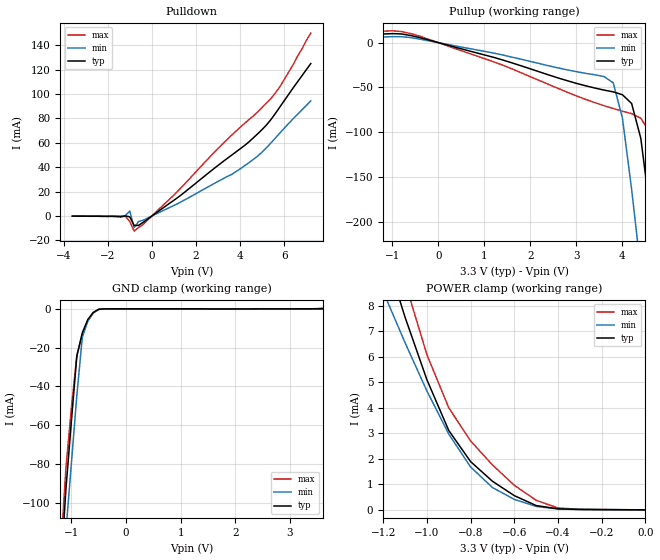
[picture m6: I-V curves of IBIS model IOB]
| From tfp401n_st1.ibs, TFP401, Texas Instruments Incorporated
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|   INPUT / OUTPUT  MODEL
[Model]   IOB
Model_type   I/O
| Signals   CTL1, CTL2, CTL3, SCDT
Vinl = 1.08
Vinh = 2.10
| variable   typ   min   max
C_comp   2pF   NA   NA
|   typ   min   max
[Temperature Range] 25.0   70.0   0.0
[Voltage range]   3.3V   3.0V   3.6V
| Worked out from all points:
|   slope of the pulldown table from 0 to 0.495 V, typ, clamps not added: 76.7 ohm
|   slope of the pullup table from 0 to 0.495 V, typ, clamps not added: 72.2 ohm
|   GND clamp passes 1 mA (typ) near -0.55 V on its own axis
|   POWER clamp passes 1 mA (typ) near -0.68 V on its own axis
[GND_clamp]
|Voltage   I(typ)   I(min)   I(max)
-3.6V     -1.31A     -1.33A     -1.29A
-1.2V     -138mA     -161mA     -127mA
-1.1V     -93mA      -115mA     -82.2mA
-1V       -58mA      -79.8mA    -51.2mA
-900mV    -24.3mA    -44.7mA    -24.1mA
-800mV    -12.4mA    -14.8mA    -13.4mA
-700mV    -5.53mA    -6.32mA    -6.36mA
-600mV    -1.83mA    -2.13mA    -2.17mA
-500mV    -221uA     -304uA     -325uA
3.3V      5.05nA     13.8uA     -16.9uA
3.6V      15.8uA     402uA      272pA
[Power_clamp]
|Note that the [Power_clamp] voltage table is referenced to Vcc
|and is calculated using Vtable=Vcc-Vmeasured.
|Voltage   I(typ)   I(min)   I(max)
-3.3V     76.1mA     54.4mA     97mA
-1.2V     10.3mA     8.55mA     12.2mA
-1.1V     7.55mA     6.55mA     8.92mA
-1V       5.1mA      4.66mA     6.08mA
-900mV    3.11mA     2.97mA     4mA
-800mV    1.89mA     1.68mA     2.7mA
-700mV    1.12mA     874uA      1.76mA
-600mV    557uA      410uA      963uA
-500mV    168uA      135uA      373uA
-400mV    40.3uA     33.2uA     73.3uA
-300mV    15.9uA     13.2uA     21.8uA
0V        146pA      221pA      155pA
[Pulldown]
|Voltage   I(typ)   I(min)   I(max)
-3.6V     -109uA     -74.8uA    -142uA
-1.2V     118uA      307uA      -179uA
-1V       -698uA     4.1mA      -4.47mA
-800mV    -7.8mA     -9.49mA    -12.4mA
-600mV    -7.64mA    -4.51mA    -9.37mA
-400mV    -5.28mA    -3.51mA    -7.03mA
1V        12.9mA     8.65mA     17.2mA
3.6V      49.7mA     33.9mA     66mA
4.8V      67.5mA     49.2mA     85.4mA
5.4V      79.2mA     60mA       96.4mA
5.8V      89.4mA     68.1mA     106mA
7.2V      125mA      94.4mA     150mA
[Pullup]
|Note that the [Pullup] voltage table is referenced to Vcc
|and is calculated using Vtable=Vcc-Vmeasured.
|Voltage   I(typ)   I(min)   I(max)
-3.2V     2.59mA     2.04mA     3.21mA
-800mV    9.73mA     6.7mA      12.4mA
1.2V      -16.4mA    -11.6mA    -21.4mA
3.6V      -53mA      -37.9mA    -70.5mA
3.8V      -55mA      -44.9mA    -73.6mA
4V        -58.2mA    -84.3mA    -76.6mA
4.2V      -68mA      -164mA     -79.4mA
4.4V      -107mA     -255mA     -84.5mA
4.6V      -188mA     -349mA     -101mA
4.8V      -280mA     -445mA     -142mA
5V        -374mA     -542mA     -223mA
6.6V      -1.16A     -1.33A     -998mA
[Ramp]
|   typ   min   max
dV/dt_r   1.95v/0.86ns   1.77v/1.32ns   2.14v/0.58ns
dV/dt_f   1.95v/0.71ns   1.76v/1.13ns   2.14v/0.45ns
R_load = 5K
